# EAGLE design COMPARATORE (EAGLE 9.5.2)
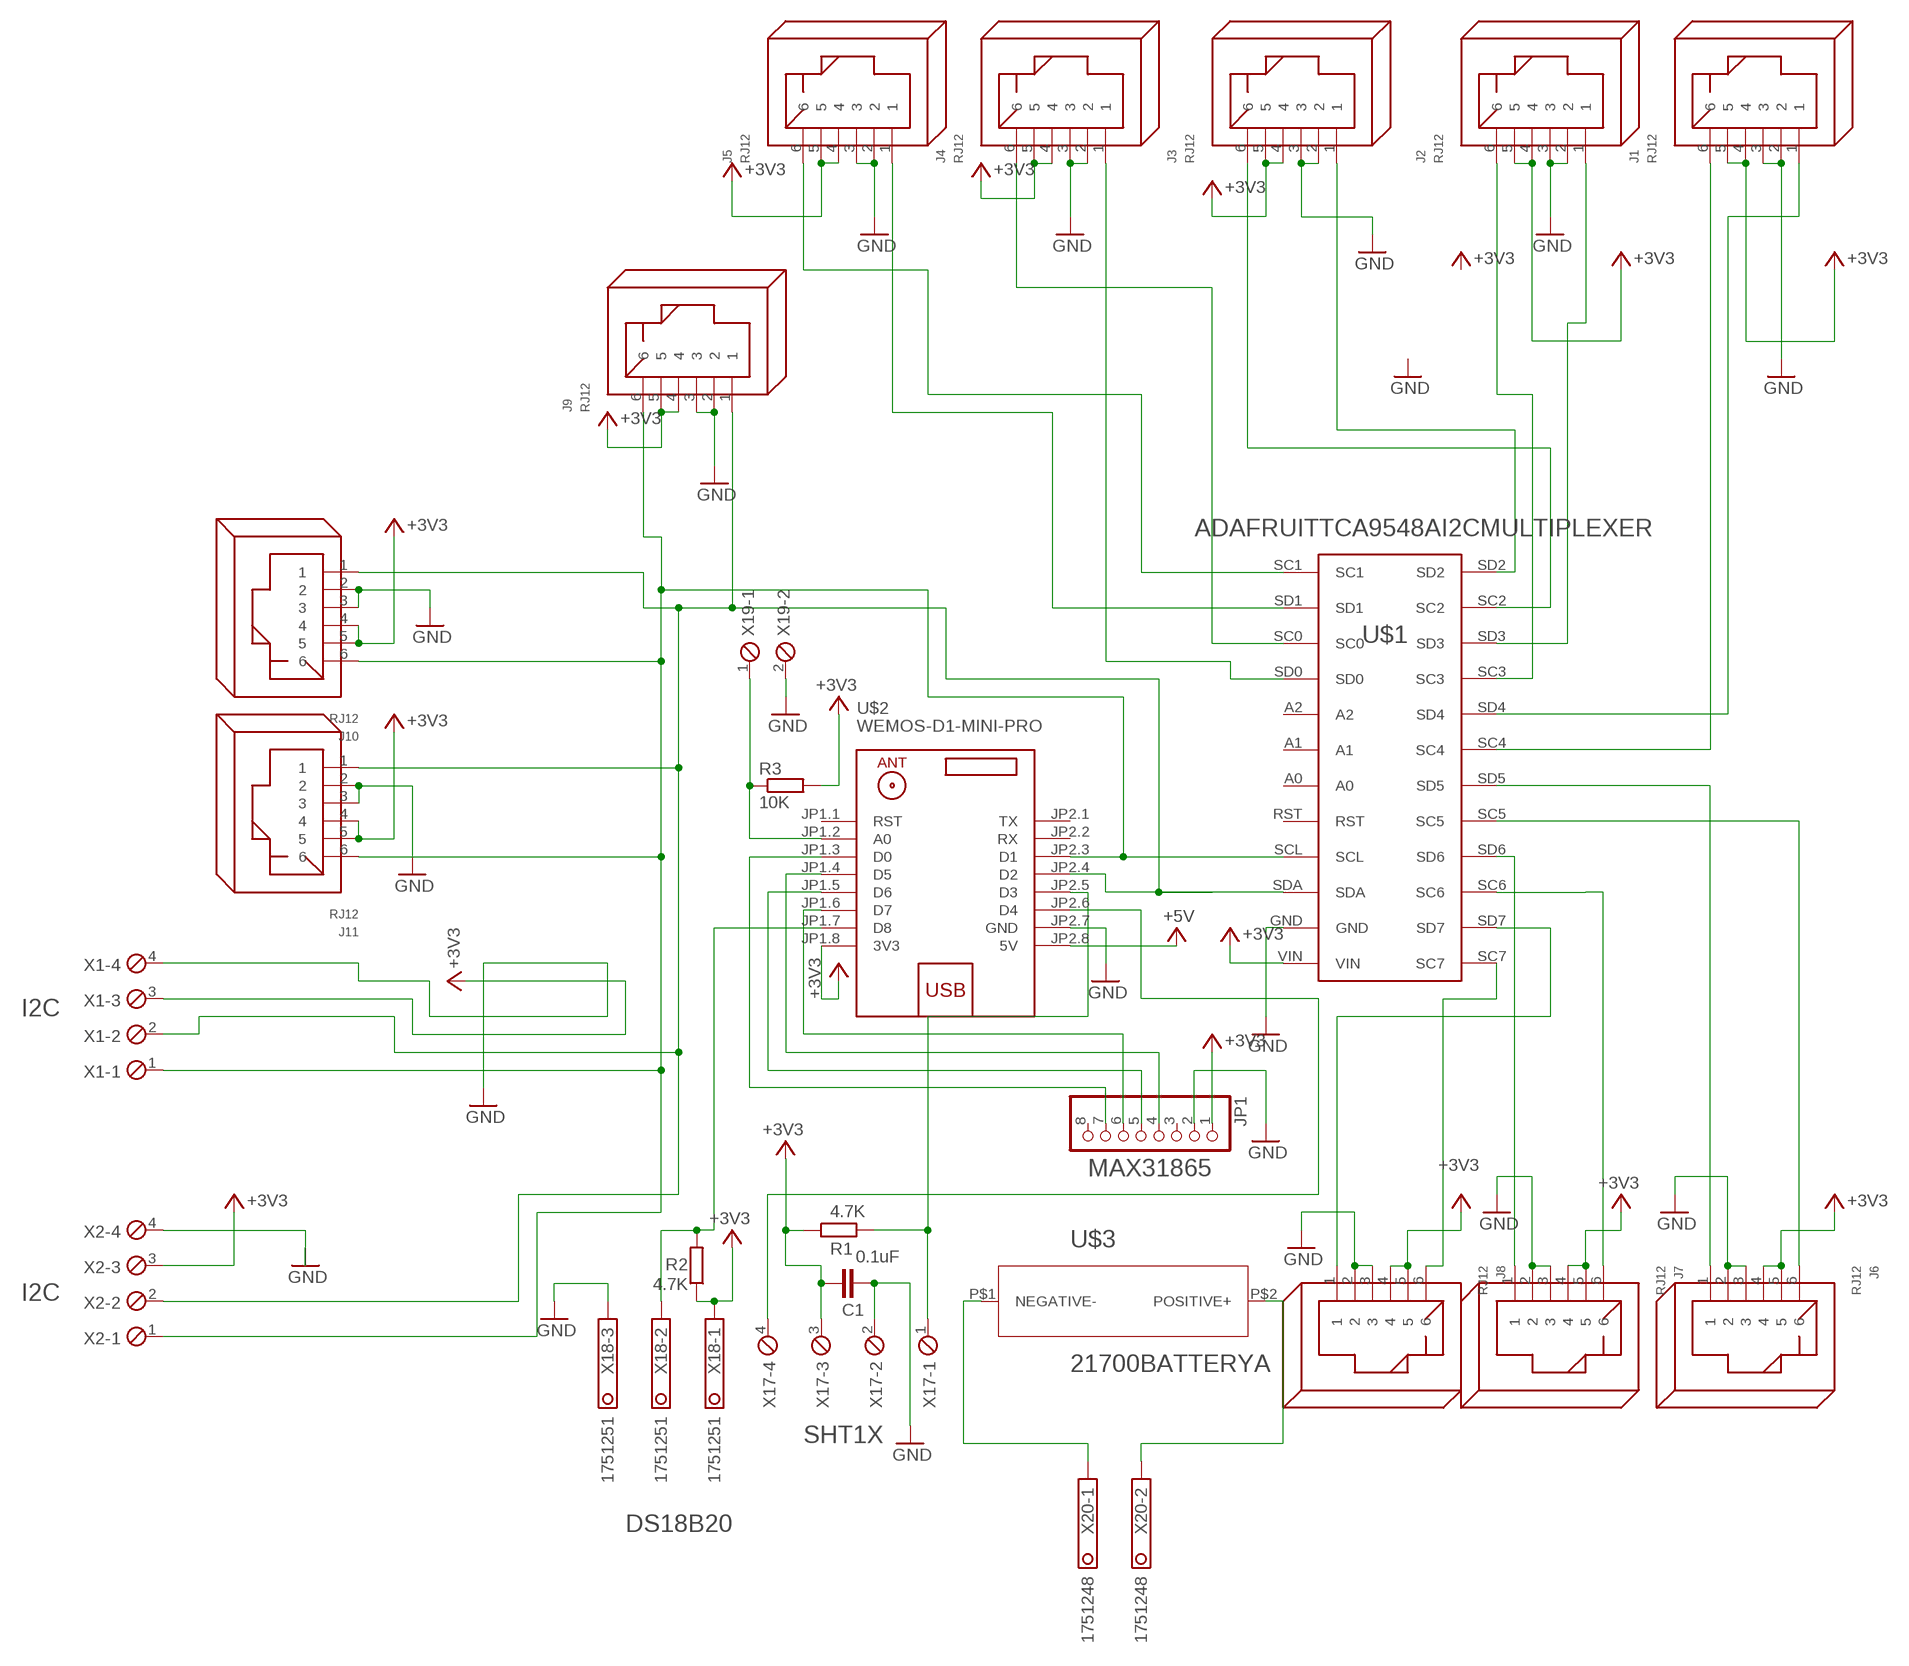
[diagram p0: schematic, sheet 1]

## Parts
C1  0.1uF  C-EUC0805  [C0805]
J1  RJ12  [RJ12]
J2  RJ12  [RJ12]
J3  RJ12  [RJ12]
J4  RJ12  [RJ12]
J5  RJ12  [RJ12]
J6  RJ12  [RJ12]
J7  RJ12  [RJ12]
J8  RJ12  [RJ12]
J9  RJ12  [RJ12]
J10  RJ12  [RJ12]
J11  RJ12  [RJ12]
JP1  PINHD-1X8  [1X08]
R1  4.7K  R-EU_R0805  [R0805]
R2  4.7K  R-EU_R0805  [R0805]
R3  10K  R-EU_R0805  [R0805]
U$1  ADAFRUITTCA9548AI2CMULTIPLEXER  [TCA9548AI2CMULTIPLEXER]
U$2  WEMOS-D1-MINI-PRO  [WEMOS-D1-MINI-PRO]
U$3  21700BATTERYA  [21700BATTERYHOLDER]
X1  MPT4  [4POL254]
X2  MPT4  [4POL254]
X17  MPT4  [4POL254]
X18  1751251  [1751251]
X19  MPT2  [2POL254]
X20  1751248  [1751248]

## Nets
+3V3: C1.1 J1.4 J1.5 J2.4 J2.5 J3.4 J3.5 J4.4 J4.5 J5.4 J5.5 J6.4 J6.5 J7.4 J7.5 J8.4 J8.5 J9.4 J9.5 J10.4 J10.5 J11.4 J11.5 JP1.1 R1.1 R2.1 R3.2 U$1.VIN U$2.JP1.8(3V3) X1.3 X2.3 X17.3 X18.1
+5V: U$2.JP2.8(5V)
CLK: JP1.4 U$2.JP1.4(D5)
CLOCK: U$2.JP2.6(D4) X17.4
CS: JP1.7 U$2.JP1.3(D0)
DATA: R1.2 U$2.JP2.5(D3) X17.1
GND: C1.2 J1.2 J1.3 J2.2 J2.3 J3.2 J3.3 J4.2 J4.3 J5.2 J5.3 J6.2 J6.3 J7.2 J7.3 J8.2 J8.3 J9.2 J9.3 J10.2 J10.3 J11.2 J11.3 JP1.2 U$1.GND U$2.JP2.7(GND) X1.4 X2.4 X17.2 X18.3 X19.2
N$2: R2.2 U$2.JP1.7(D8) X18.2
N$3: R3.1 U$2.JP1.2(A0) X19.1
NEGATIVE: U$3.P$1(NEGATIVE-) X20.1
POSITIVE: U$3.P$2(POSITIVE+) X20.2
SC0: J4.6 U$1.SC0
SC1: J5.6 U$1.SC1
SC2: J3.6 U$1.SC2
SC3: J2.6 U$1.SC3
SC4: J1.6 U$1.SC4
SC5: J6.6 U$1.SC5
SC6: J7.6 U$1.SC6
SC7: J8.6 U$1.SC7
SCL: J9.6 J10.6 J11.6 U$1.SCL U$2.JP2.3(D1) X1.1 X2.1
SD0: J4.1 U$1.SD0
SD1: J5.1 U$1.SD1
SD2: J3.1 U$1.SD2
SD3: J2.1 U$1.SD3
SD4: J1.1 U$1.SD4
SD5: J6.1 U$1.SD5
SD6: J7.1 U$1.SD6
SD7: J8.1 U$1.SD7
SDA: J9.1 J10.1 J11.1 U$1.SDA U$2.JP2.4(D2) X1.2 X2.2
SDI: JP1.6 U$2.JP1.6(D7)
SDO: JP1.5 U$2.JP1.5(D6)
Unconnected: JP1.3 JP1.8 U$1.A0 U$1.A1 U$1.A2 U$1.RST U$2.JP1.1(RST) U$2.JP2.1(TX) U$2.JP2.2(RX)

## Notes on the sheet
- I2C
- MAX31865
- I2C
- SHT1X
- DS18B20

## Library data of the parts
C1 = rcl:C-EU: CAPACITOR, European symbol; SPICEPREFIX: C
J1-J11 = con-rj:RJ12: RJ12, RJ14 and RJ25 RJ12, RJ14 and RJ25 jacks side mounted http://www.tycoelectronics.com
JP1 = pinhead:PINHD-1X8: PIN HEADER
R1-R3 = rcl:R-EU_: RESISTOR, European symbol; SPICEPREFIX: R
U$1 = TCA9548AI2CMultiplexer:ADAFRUITTCA9548AI2CMULTIPLEXER
U$2 = diy-modules:WEMOS-D1-MINI-PRO: WEMOS D1 mini Pro: Mini Wi-Fi Board based on ESP-8266EX chip More details can be found here: https://www.wemos.cc/product/d1-mini-pro.html Click here to find device on ebay.com
U$3 = LithiumBatteryHolder21700:21700BATTERY
X1 X2 X17 = con-phoenix-254:MPT4: PHOENIX CONNECTOR; OC_FARNELL: unknown; OC_NEWARK: unknown
X18 = con-phoenix-350:1751251: MKDS 1/ 3-3,5 Printklemme Nennstrom: 10 A Bemessungsspannung: 160 V Raster: 3,5 mm Polzahl: 3 Montageart: Löten Anschlussart: Schraubanschluss Anschlussrichtung vom Leiter zur Platine: 0° Source: http://eshop.phoenixcontact.com .. 1751251.pdf; OC_FARNELL: unknown; OC_NEWARK: unknown
X19 = con-phoenix-254:MPT2: PHOENIX CONNECTOR; OC_FARNELL: unknown; OC_NEWARK: unknown
X20 = con-phoenix-350:1751248: MKDS 1/ 2-3,5 Printklemme; OC_FARNELL: unknown; OC_NEWARK: unknown

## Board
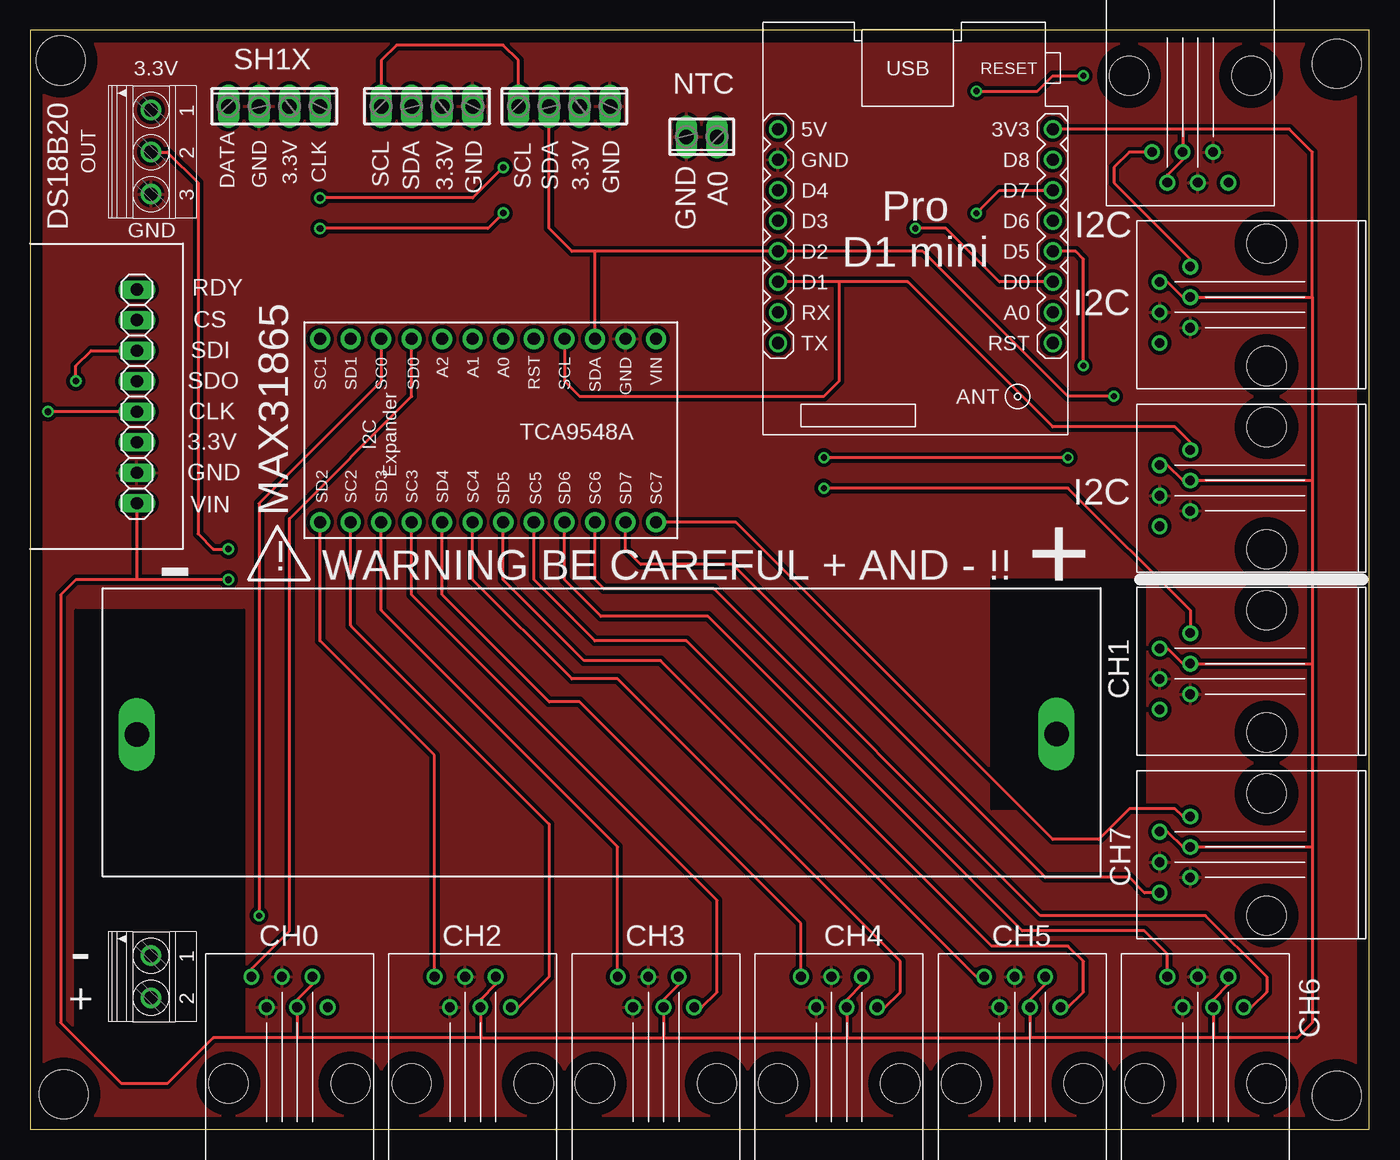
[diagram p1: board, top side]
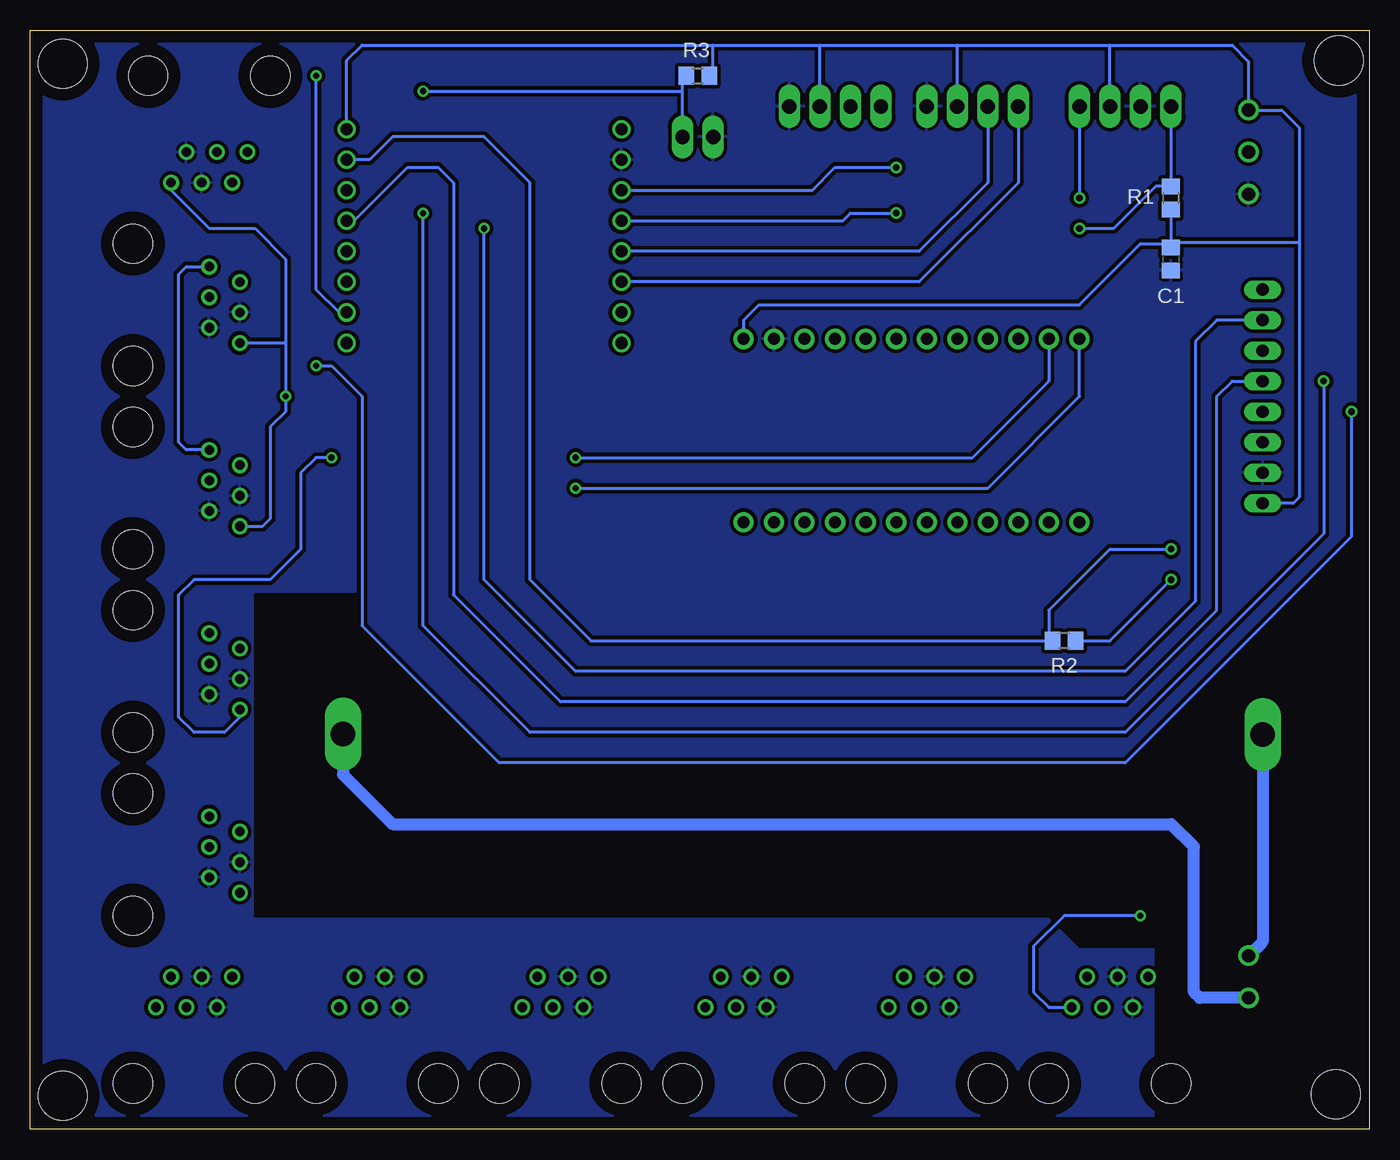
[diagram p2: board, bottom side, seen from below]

Size 111.43 x 91.43 mm. Coordinates in mm from the lower left corner, seen from the top.
Outline: 0,0 111.43,0 111.43,91.43 0,91.43 0,0
Copper layers (1*16): Top 0.035mm / dielectric 1.5mm / Bottom 0.035mm
Design rules "default": minimum track width 6mil, minimum drill 0.35mm, track to track 6mil, track to pad 6mil, pad to pad 6mil, via to via 6mil, smd to smd 6mil, copper to edge 40mil, drill to drill 6mil, minimum pad ring 10mil, minimum via ring 8mil, stop-mask expansion 4mil, vias tented up to drill 0mil, thermal gap 10mil
Holes 4.06 mm at 2.54,88.9 108.71,88.65 108.71,2.79 2.79,2.92

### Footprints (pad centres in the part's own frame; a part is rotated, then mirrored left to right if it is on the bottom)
C0805 = smd 1.3 x 1.5: 1 -0.95,0; 2 0.95,0
RJ12 = drill 0.8: 1 -8.89,-3.175; 2 -6.35,-1.905; 3 -8.89,-0.635; 4 -6.35,0.635; 5 -8.89,1.905; 6 -6.35,3.175 | hole 3.25: 0,-5.08; 0,5.08
1X08 = drill 1.016 long: 1 -8.89,0; 2 -6.35,0; 3 -3.81,0; 4 -1.27,0; 5 1.27,0; 6 3.81,0; 7 6.35,0; 8 8.89,0
R0805 = smd 1.3 x 1.5: 1 -0.95,0; 2 0.95,0
TCA9548AI2CMULTIPLEXER = drill 1 pad 1.676: A0 -8.59,2.54; A1 -8.59,0; A2 -8.59,-2.54; GND -8.59,12.7; RST -8.59,5.08; SC0 -8.59,-7.62; SC1 -8.59,-12.7; SC2 6.65,-10.16; SC3 6.65,-5.08; SC4 6.65,0; SC5 6.65,5.08; SC6 6.65,10.16; SC7 6.65,15.24; SCL -8.59,7.62; SD0 -8.59,-5.08; SD1 -8.59,-10.16; SD2 6.65,-12.7; SD3 6.65,-7.62; SD4 6.65,-2.54; SD5 6.65,2.54; SD6 6.65,7.62; SD7 6.65,12.7; SDA -8.59,10.16; VIN -8.59,15.24
WEMOS-D1-MINI-PRO = drill 1: JP1.1 -11.43,9.525; JP1.2 -11.43,6.985; JP1.3 -11.43,4.445; JP1.4 -11.43,1.905; JP1.5 -11.43,-0.635; JP1.6 -11.43,-3.175; JP1.7 -11.43,-5.715; JP1.8 -11.43,-8.255; JP2.1 11.43,9.525; JP2.2 11.43,6.985; JP2.3 11.43,4.445; JP2.4 11.43,1.905; JP2.5 11.43,-0.635; JP2.6 11.43,-3.175; JP2.7 11.43,-5.715; JP2.8 11.43,-8.255
21700BATTERYHOLDER = drill 2.032 long: P$1 -11.43,-0.171; P$2 65.07,-0.127
4POL254 = drill 1.2 long: 1 -3.81,0; 2 -1.27,0; 3 1.27,0; 4 3.81,0
1751251 = drill 1.1 pad 1.7: 1 -3.5,-0.1; 2 0,-0.1; 3 3.5,-0.1
2POL254 = drill 1.2 long: 1 -1.27,0; 2 1.27,0
1751248 = drill 1.1 pad 1.7: 1 -1.75,-0.1; 2 1.75,-0.1

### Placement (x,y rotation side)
C1  16.51,72.39 270 bottom
J1  67.31,3.81 270 top
J2  52.07,3.81 270 top
J3  36.83,3.81 270 top
J4  21.59,3.81 270 top
J5  102.87,38.1 0 top
J6  82.55,3.81 270 top
J7  97.79,3.81 270 top
J8  102.87,22.86 0 top
J9  102.87,53.34 0 top
J10  102.87,68.58 0 top
J11  96.52,87.63 90 top
JP1  8.89,60.96 90 top
R1  16.51,77.47 90 bottom
R2  25.4,40.64 180 bottom
R3  55.88,87.63 0 bottom
U$1  36.83,57.15 270 top
U$2  73.66,74.93 180 top
U$3  20.32,33.02 0 top
X1  44.45,85.09 0 top
X2  33.02,85.09 0 top
X17  20.32,85.09 0 top
X18  10.16,81.28 270 top
X19  55.88,82.55 180 top
X20  10.16,12.7 270 top

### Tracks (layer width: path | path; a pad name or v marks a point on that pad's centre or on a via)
+3V3  (via drill 0.55)
  Top 0.254: 37.47,7.62 22.23,7.62 | 37.47,7.62 52.7,7.62 | 52.7,7.62 67.94,7.62 | 67.94,7.62 83.19,7.62 | v16.51,45.72 8.89,45.72 | 67.94,7.62 J1.4 67.94,10.79 69.22,12.07 J1.5 | 22.23,7.62 J4.4 22.23,10.79 23.5,12.07 J4.5 | 37.47,7.62 J3.4 37.47,10.79 38.73,12.07 J3.5 | 52.7,7.62 J2.4 52.7,10.79 53.98,12.07 J2.5 | 83.19,7.62 J6.4 83.19,10.79 84.45,12.07 J6.5 | 106.68,69.22 106.68,53.97 | 106.68,53.97 106.68,38.73 | 106.68,38.73 106.68,23.5 | 106.68,23.5 106.68,8.89 105.41,7.62 98.42,7.62 | 98.42,7.62 83.19,7.62 | 98.42,7.62 J7.4 98.42,10.79 99.7,12.07 J7.5 | 106.68,23.5 J8.4 95.89,23.5 94.61,24.77 J8.5 | 106.68,53.97 J9.4 95.89,53.97 94.61,55.24 J9.5 | 95.89,83.19 U$2.JP1.8 | 95.89,83.19 J11.4 95.89,80.65 94.61,79.38 J11.5 | 106.68,69.22 J10.4 95.89,69.22 94.61,70.48 J10.5 | 106.68,38.73 J5.4 95.89,38.73 94.61,40 J5.5 | 95.89,83.19 104.78,83.19 106.68,81.28 106.68,69.22 | 22.23,7.62 15.24,7.62 11.43,3.81 7.62,3.81 2.54,8.89 2.54,44.45 3.81,45.72 8.89,45.72 | JP1.1 8.89,45.72
  Bottom 0.254: U$2.JP1.8 85.09,88.9 83.82,90.17 54.61,90.17 | 5.84,73.79 16.51,73.79 R1.1 16.51,73.66 | 16.51,73.66 C1.1 | U$1.VIN 52.07,67.31 50.8,68.58 24.13,68.58 19.05,73.66 16.51,73.66 | 54.61,90.17 45.72,90.17 | 45.72,90.17 34.29,90.17 | 34.29,90.17 21.59,90.17 | X17.3 21.59,90.17 | X2.3 34.29,90.17 | X1.3 45.72,90.17 | R2.1 21.59,40.64 v16.51,45.72 | R3.2 54.61,87.95 54.61,90.17 | 5.84,73.79 5.84,83.31 7.31,84.78 X18.1 10.06,88.8 11.43,90.17 21.59,90.17 | 5.84,73.79 5.84,52.58 6.35,52.07 JP1.1
CLK  (via drill 0.51, 0.55)
  Top 0.254: JP1.4 v1.49,59.69 | U$2.JP1.4 87,73.03 87.63,72.39 v87.63,63.5
  Bottom 0.254: v1.49,59.69 1.49,49.31 20.32,30.48 72.39,30.48 83.82,41.91 83.82,60.96 86.36,63.5 v87.63,63.5
CLOCK  (via drill 0.55)
  Top 0.254: v39.37,80.01 36.83,77.47 v24.13,77.47
  Bottom 0.254: X17.4 v24.13,77.47 | U$2.JP2.6 46.36,78.11 44.45,80.01 v39.37,80.01
CS  (via drill 0.51)
  Top 0.254: U$2.JP1.3 80.64,70.48 76.2,74.93 v73.66,74.93
  Bottom 0.254: JP1.7 12.7,67.31 14.48,65.53 14.48,43.94 20.32,38.1 66.04,38.1 73.66,45.72 v73.66,74.93
DATA  (via drill 0.55)
  Top 0.254: v39.37,76.2 38.1,74.93 v24.13,74.93
  Bottom 0.254: X17.1 R1.2 17.78,78.42 21.27,74.93 v24.13,74.93 | U$2.JP2.5 43.81,75.56 43.18,76.2 v39.37,76.2
GND
  pour Top (isolate 0.305, rank 2): 0,91.44 111.76,91.44 111.76,0 0,0
  pour Bottom (isolate 0.305, rank 2): 0,91.44 111.76,91.44 111.76,0 0,0
N$2  (via drill 0.55)
  Top 0.254: X18.2 11.43,81.28 13.97,78.74 13.97,49.53 15.24,48.26 v16.51,48.26
  Bottom 0.254: 26.67,40.64 64.77,40.64 69.85,45.72 69.85,78.74 73.66,82.55 81.28,82.55 83.19,80.65 U$2.JP1.7 | 26.67,40.64 R2.2 | 26.67,40.64 26.67,43.18 21.59,48.26 v16.51,48.26
N$3  (via drill 0.51)
  Top 0.254: v78.74,86.36 83.82,86.36 85.09,87.63 v87.63,87.63
  Bottom 0.254: U$2.JP1.2 85.72,67.95 87.63,69.85 v87.63,87.63 | v78.74,86.36 57.15,86.36 | R3.1 57.15,87.63 57.15,86.36 | X19.1 57.15,86.36
NEGATIVE
  Bottom 1.016: U$3.P$1 8.89,15.62 X20.1
  cutout Top: 3.81,43.18 17.78,43.18 17.78,7.62 3.81,7.62
  cutout Bottom: 17.78,12.7 17.78,0 0,0 0,35.56 15.24,35.56 17.78,33.02
POSITIVE
  Bottom 1.016: X20.2 14.12,10.95 14.61,11.43 14.61,23.5 16.51,25.4 81.28,25.4 85.39,29.51 U$3.P$2
  cutout Top (isolate 2.184): 80.01,45.72 92.71,45.72 92.71,26.67 80.01,26.67
  cutout Bottom (isolate 0.305): 17.78,15.24 17.78,30.48 83.82,30.48 83.82,44.45 92.71,44.45 92.71,17.78 26.67,17.78 24.13,15.24
SC0  (via drill 0.51)
  Top 0.254: U$1.SC0 29.21,62.23 19.05,52.07 v19.05,17.78
  Bottom 0.254: v19.05,17.78 25.4,17.78 27.94,15.24 27.94,11.43 26.67,10.16 J4.6
SC1  (via drill 0.51)
  Top 0.254: J5.6 96.52,43.18 86.36,53.34 v66.04,53.34
  Bottom 0.254: U$1.SC1 24.13,60.96 31.75,53.34 v66.04,53.34
SC2
  Top 0.254: J3.6 40.64,10.16 43.18,12.7 43.18,25.4 26.67,41.91 U$1.SC2
SC3
  Top 0.254: J2.6 55.88,10.16 57.15,11.43 57.15,19.05 31.75,44.45 U$1.SC3
SC4
  Top 0.254: J1.6 71.12,10.16 72.39,11.43 72.39,13.97 48.9,37.46 45.09,37.46 36.83,45.72 U$1.SC4
SC5
  Top 0.254: J6.6 86.36,10.16 87.63,11.43 87.63,13.97 86.36,15.24 80.01,15.24 54.61,40.64 46.99,40.64 41.91,45.72 U$1.SC5
SC6
  Top 0.254: J7.6 101.6,10.16 102.87,11.43 102.87,12.7 97.79,17.78 84.07,17.78 56.9,44.96 47.75,44.96 46.99,45.72 U$1.SC6
SC7
  Top 0.254: J8.6 95.89,26.04 95.25,26.67 91.44,26.67 88.9,24.13 85.09,24.13 58.72,50.5 U$1.SC7
SCL
  Top 0.254: 67.31,70.48 73.03,70.48 85.09,58.42 95.25,58.42 96.52,57.15 J9.6 | 67.31,70.48 U$2.JP2.3 | 67.31,70.48 67.31,62.23 66.04,60.96 45.72,60.96 44.45,62.23 U$1.SCL | J11.6 91.44,81.28 90.17,80.01 90.17,78.74 96.52,72.39 J10.6 | X1.1 40.64,88.9 39.37,90.17 30.48,90.17 29.21,88.9 X2.1
  Bottom 0.254: X2.1 29.21,78.74 37.47,70.48 U$2.JP2.3 | J9.6 98.42,56.52 99.06,57.15 99.06,71.12 98.42,71.76 J10.6
SD0
  Top 0.254: U$1.SD0 31.75,60.96 21.59,50.8 21.59,16.51 18.41,13.34 J4.1
SD1  (via drill 0.51)
  Top 0.254: v86.36,55.88 v66.04,55.88
  Bottom 0.254: v66.04,55.88 33.02,55.88 26.67,62.23 U$1.SD1 | v86.36,55.88 87.63,55.88 88.9,54.61 88.9,48.26 91.44,45.72 97.79,45.72 99.06,44.45 99.06,34.29 97.79,33.02 95.25,33.02 93.98,34.29 J5.1
SD2
  Top 0.254: J3.1 33.66,31.12 24.13,40.64 U$1.SD2
SD3
  Top 0.254: J2.1 48.9,23.5 29.21,43.18 U$1.SD3
SD4
  Top 0.254: U$1.SD4 34.29,44.45 43.18,35.56 45.72,35.56 64.13,17.14 J1.1
SD5
  Top 0.254: U$1.SD5 39.37,45.72 46.1,38.99 52.45,38.99 78.74,12.7 J6.1
SD6
  Top 0.254: J7.1 94.61,14.61 92.71,16.51 82.55,16.51 56.39,42.67 47.5,42.67 44.45,45.72 U$1.SD6
SD7
  Top 0.254: J8.1 92.71,19.68 91.44,20.96 84.45,20.96 58.42,46.99 50.8,46.99 49.53,48.26 U$1.SD7
SDA  (via drill 0.51)
  Top 0.254: 46.99,73.03 U$2.JP2.4 74.3,73.03 86.36,60.96 v90.17,60.96 | U$1.SDA 46.99,73.03 | 46.99,73.03 45.09,73.03 43.18,74.93 X1.2
  Bottom 0.254: X2.2 31.75,78.74 37.47,73.03 U$2.JP2.4 | J9.1 92.08,50.16 91.44,50.8 91.44,58.42 90.17,59.69 v90.17,60.96 90.17,65.41 | J11.1 99.7,78.11 96.52,74.93 92.71,74.93 90.17,72.39 90.17,65.41 | J10.1 90.17,65.41
SDI  (via drill 0.51, 0.55)
  Top 0.254: v78.74,76.2 80.64,78.11 U$2.JP1.6 | v3.81,62.23 3.81,63.5 5.08,64.77 JP1.6
  Bottom 0.254: v3.81,62.23 3.81,49.53 20.32,33.02 69.85,33.02 78.74,41.91 v78.74,76.2
SDO
  Bottom 0.254: U$2.JP1.5 84.45,75.56 80.01,80.01 77.47,80.01 76.2,78.74 76.2,44.45 67.31,35.56 20.32,35.56 12.7,43.18 12.7,60.96 11.43,62.23 JP1.5

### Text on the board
tPlace: SH1X | 3.3V | NTC | GND | OUT | DATA | 3.3V | CLK | SCL | SCL | SDA | 3.3V | GND | SDA | 3.3V | GND | A0 | DS18B20 | GND | GND | I2C | RDY | I2C | CS | SDI | SDO | CLK | 3.3V | GND | VIN | I2C | MAX31865 | ! | WARNING BE CAREFUL + AND - !! | + | - | CH1 | CH7 | CH0 | CH2 | CH3 | CH4 | CH5 | - | + | CH6

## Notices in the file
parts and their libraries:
diy-modules: Released under the Creative Commons Attribution 4.0 International License: http://creativecommons.org/licenses/by/4.0
